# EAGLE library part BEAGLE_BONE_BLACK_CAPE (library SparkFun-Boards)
BeagleBone Black Rev C Cape Generic footprint for BeagleBone Black Rev C Capes. SparkFun Products: SparkFun BeagleBone Black Proto Cape SparkFun CryptoCape
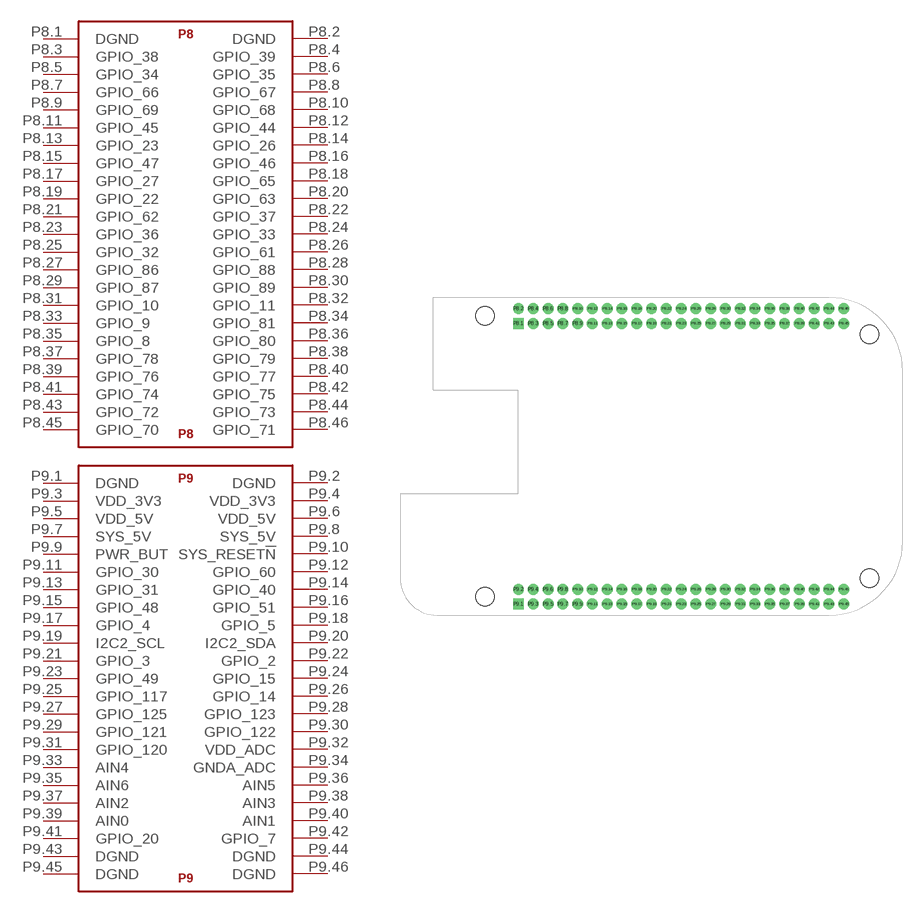
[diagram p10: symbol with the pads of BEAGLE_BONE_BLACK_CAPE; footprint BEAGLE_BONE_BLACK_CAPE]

Designator prefix B; gates P8=BEAGLE_BONE_BLACK_P8 P9=BEAGLE_BONE_BLACK_P9

## BEAGLE_BONE_BLACK_CAPE  [BEAGLE_BONE_BLACK_CAPE]
P8.1  P8:DGND
P8.2  P8:DGND
P8.3  P8:GPIO_38
P8.4  P8:GPIO_39
P8.5  P8:GPIO_34
P8.6  P8:GPIO_35
P8.7  P8:GPIO_66
P8.8  P8:GPIO_67
P8.9  P8:GPIO_69
P8.10  P8:GPIO_68
P8.11  P8:GPIO_45
P8.12  P8:GPIO_44
P8.13  P8:GPIO_23
P8.14  P8:GPIO_26
P8.15  P8:GPIO_47
P8.16  P8:GPIO_46
P8.17  P8:GPIO_27
P8.18  P8:GPIO_65
P8.19  P8:GPIO_22
P8.20  P8:GPIO_63
P8.21  P8:GPIO_62
P8.22  P8:GPIO_37
P8.23  P8:GPIO_36
P8.24  P8:GPIO_33
P8.25  P8:GPIO_32
P8.26  P8:GPIO_61
P8.27  P8:GPIO_86
P8.28  P8:GPIO_88
P8.29  P8:GPIO_87
P8.30  P8:GPIO_89
P8.31  P8:GPIO_10
P8.32  P8:GPIO_11
P8.33  P8:GPIO_9
P8.34  P8:GPIO_81
P8.35  P8:GPIO_8
P8.36  P8:GPIO_80
P8.37  P8:GPIO_78
P8.38  P8:GPIO_79
P8.39  P8:GPIO_76
P8.40  P8:GPIO_77
P8.41  P8:GPIO_74
P8.42  P8:GPIO_75
P8.43  P8:GPIO_72
P8.44  P8:GPIO_73
P8.45  P8:GPIO_70
P8.46  P8:GPIO_71
P9.1  P9:DGND
P9.2  P9:DGND
P9.3  P9:VDD_3V3
P9.4  P9:VDD_3V3
P9.5  P9:VDD_5V
P9.6  P9:VDD_5V
P9.7  P9:SYS_5V
P9.8  P9:SYS_5V
P9.9  P9:PWR_BUT
P9.10  P9:SYS_RESET!N
P9.11  P9:GPIO_30
P9.12  P9:GPIO_60
P9.13  P9:GPIO_31
P9.14  P9:GPIO_40
P9.15  P9:GPIO_48
P9.16  P9:GPIO_51
P9.17  P9:GPIO_4
P9.18  P9:GPIO_5
P9.19  P9:I2C2_SCL
P9.20  P9:I2C2_SDA
P9.21  P9:GPIO_3
P9.22  P9:GPIO_2
P9.23  P9:GPIO_49
P9.24  P9:GPIO_15
P9.25  P9:GPIO_117
P9.26  P9:GPIO_14
P9.27  P9:GPIO_125
P9.28  P9:GPIO_123
P9.29  P9:GPIO_121
P9.30  P9:GPIO_122
P9.31  P9:GPIO_120
P9.32  P9:VDD_ADC
P9.33  P9:AIN4
P9.34  P9:GNDA_ADC
P9.35  P9:AIN6
P9.36  P9:AIN5
P9.37  P9:AIN2
P9.38  P9:AIN3
P9.39  P9:AIN0
P9.40  P9:AIN1
P9.41  P9:GPIO_20
P9.42  P9:GPIO_7
P9.43  P9:DGND
P9.44  P9:DGND
P9.45  P9:DGND
P9.46  P9:DGND

## Footprint BEAGLE_BONE_BLACK_CAPE (pad centres in mm)
drill 1.016 pad 1.88 square: P8.1 20.32,50.165; P9.1 20.32,1.905
drill 1.016 pad 1.88: P8.2 20.32,52.705; P8.3 22.86,50.165; P8.4 22.86,52.705; P8.5 25.4,50.165; P8.6 25.4,52.705; P8.7 27.94,50.165; P8.8 27.94,52.705; P8.9 30.48,50.165; P8.10 30.48,52.705; P8.11 33.02,50.165; P8.12 33.02,52.705; P8.13 35.56,50.165; P8.14 35.56,52.705; P8.15 38.1,50.165; P8.16 38.1,52.705; P8.17 40.64,50.165; P8.18 40.64,52.705; P8.19 43.18,50.165; P8.20 43.18,52.705; P8.21 45.72,50.165; P8.22 45.72,52.705; P8.23 48.26,50.165; P8.24 48.26,52.705; P8.25 50.8,50.165; P8.26 50.8,52.705; P8.27 53.34,50.165; P8.28 53.34,52.705; P8.29 55.88,50.165; P8.30 55.88,52.705; P8.31 58.42,50.165; P8.32 58.42,52.705; P8.33 60.96,50.165; P8.34 60.96,52.705; P8.35 63.5,50.165; P8.36 63.5,52.705; P8.37 66.04,50.165; P8.38 66.04,52.705; P8.39 68.58,50.165; P8.40 68.58,52.705; P8.41 71.12,50.165; P8.42 71.12,52.705; P8.43 73.66,50.165; P8.44 73.66,52.705; P8.45 76.2,50.165; P8.46 76.2,52.705; P9.2 20.32,4.445; P9.3 22.86,1.905; P9.4 22.86,4.445; P9.5 25.4,1.905; P9.6 25.4,4.445; P9.7 27.94,1.905; P9.8 27.94,4.445; P9.9 30.48,1.905; P9.10 30.48,4.445; P9.11 33.02,1.905; P9.12 33.02,4.445; P9.13 35.56,1.905; P9.14 35.56,4.445; P9.15 38.1,1.905; P9.16 38.1,4.445; P9.17 40.64,1.905; P9.18 40.64,4.445; P9.19 43.18,1.905; P9.20 43.18,4.445; P9.21 45.72,1.905; P9.22 45.72,4.445; P9.23 48.26,1.905; P9.24 48.26,4.445; P9.25 50.8,1.905; P9.26 50.8,4.445; P9.27 53.34,1.905; P9.28 53.34,4.445; P9.29 55.88,1.905; P9.30 55.88,4.445; P9.31 58.42,1.905; P9.32 58.42,4.445; P9.33 60.96,1.905; P9.34 60.96,4.445; P9.35 63.5,1.905; P9.36 63.5,4.445; P9.37 66.04,1.905; P9.38 66.04,4.445; P9.39 68.58,1.905; P9.40 68.58,4.445; P9.41 71.12,1.905; P9.42 71.12,4.445; P9.43 73.66,1.905; P9.44 73.66,4.445; P9.45 76.2,1.905; P9.46 76.2,4.445
hole 3.175 at 14.605,3.175
hole 3.175 at 80.645,6.35
hole 3.175 at 80.645,48.26
hole 3.175 at 14.605,51.435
